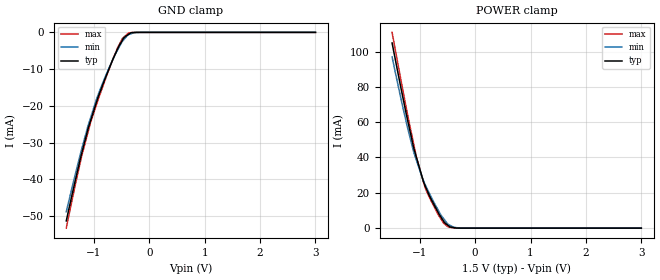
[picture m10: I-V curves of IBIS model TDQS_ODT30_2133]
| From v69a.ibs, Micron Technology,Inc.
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| MODEL TDQS_ODT30_2133 (Termination Model with 30ohm ODT, 1866/2133 Mbps)
[Model]   TDQS_ODT30_2133
Model_type   Terminator
|   typ   min   max
C_comp   1.19pF   1.04pF   1.35pF
| Note: C_comp changes when the ODT circuit is enabled.
[Voltage Range]   1.5000V   1.4250V   1.5750V
| Junction Temperature (Ambient temp is 35C typ, 95C min, 0C max)
[Temperature Range]   50.0   110.0   0.0
[Add Submodel]
| Submodel Name   Mode
30ohm_ODT_2133   Non-Driving
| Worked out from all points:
|   GND clamp passes 1 mA (typ) near -0.42 V on its own axis
|   POWER clamp passes 1 mA (typ) near -0.47 V on its own axis
[GND Clamp]
|   Voltage   I(typ)   I(min)   I(max)
-1.5V     -51.33mA   -48.85mA   -53.31mA
-1.225V   -33.17mA   -31.96mA   -33.91mA
-1.11V    -26.38mA   -25.59mA   -27.31mA
-1.06V    -24mA      -23.21mA   -24.46mA
-955mV    -19.04mA   -18.24mA   -19.74mA
-855mV    -14.8mA    -14.26mA   -15.35mA
-575mV    -4.569mA   -4.842mA   -4.255mA
-455mV    -1.373mA   -1.876mA   -1.232mA
-380mV    -600.5uA   -637.3uA   -211uA
-330mV    -105.7uA   -382.3uA   -79.03uA
-165mV    -2.061uA   -3.044uA   0A
3V        0A         0A         0A
[POWER Clamp]
|   Voltage   I(typ)   I(min)   I(max)
-1.5V     104.9mA    96.95mA    110.8mA
-1.305V   73.96mA    68.35mA    78.05mA
-1.11V    45.47mA    43.15mA    47.59mA
-1.06V    40.01mA    38.39mA    40.06mA
-955mV    28.63mA    28.51mA    28.54mA
-905mV    24.01mA    24.84mA    23.06mA
-660mV    8.35mA     9.771mA    7.255mA
-570mV    3.953mA    5.39mA     2.853mA
-490mV    1.557mA    2.191mA    712uA
-385mV    314.2uA    439.4uA    73.92uA
-265mV    10.67uA    38.19uA    0A
3V        0A         0A         0A
